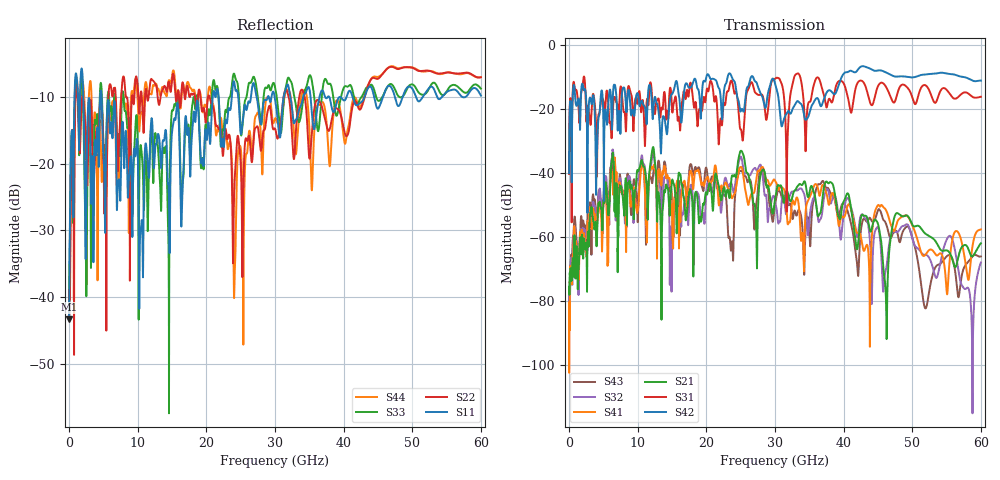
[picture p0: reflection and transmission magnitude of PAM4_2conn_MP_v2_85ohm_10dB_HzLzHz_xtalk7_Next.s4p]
! Info: Touchstone file created by Circ.  Input file=FAB50GbE_2conn_Midplane_Examax_Topo2_v2_85ohm_10dB_HzLzHz.circ
# Hz S RI R 50
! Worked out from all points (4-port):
!   6000 points, 10 MHz to 60 GHz, reference 50 ohm
!   strongest paths, dB at 10 MHz, 15.01 GHz, 30.01 GHz, 45.01 GHz, 60 GHz:
!     S42: -40.1, -15.4, -12.0, -8.0, -11.2
!     S31: -40.3, -20.3, -10.6, -12.9, -16.2
!     S21: -75.6, -42.3, -48.3, -55.9, -62.0
!     S41: -87.9, -53.9, -42.4, -50.1, -57.7
!     S32: -82.5, -57.5, -48.7, -57.0, -68.0
!     S43: -77.3, -47.4, -49.8, -51.7, -66.1
!   lowest |S11| = -43.4 dB at 10 MHz (marker M1), VSWR 1.01, Z = 50.7 - j0.0778 ohm
!   |S11| at or under -10 dB: 2.083 GHz to 4.532 GHz (2.449 GHz wide, 74 % of centre); 4.733 GHz to 20.93 GHz (16.2 GHz wide, 126 % of centre); 21.79 GHz to 23.71 GHz (1.921 GHz wide, 8.45 % of centre)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
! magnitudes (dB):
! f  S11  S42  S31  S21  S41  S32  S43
! 10 MHz  -43.4  -40.1  -40.3  -75.6  -87.9  -82.5  -77.3
! 1.1 GHz  -6.9  -19.1  -14.3  -62.9  -63.7  -61.4  -61.4
! 6.29 GHz  -15.8  -23.2  -25.3  -35.4  -40.1  -34.1  -36.8
! 24.12 GHz  -8.0  -11.5  -15.2  -40.7  -46.4  -45.0  -49.4
! 46.15 GHz  -8.8  -8.6  -13.0  -77.9  -51.5  -70.5  -55.7
! 47.76 GHz  -11.0  -9.9  -15.8  -52.5  -55.7  -58.5  -58.4
! 60 GHz  -9.8  -11.2  -16.2  -62.0  -57.7  -68.0  -66.1
